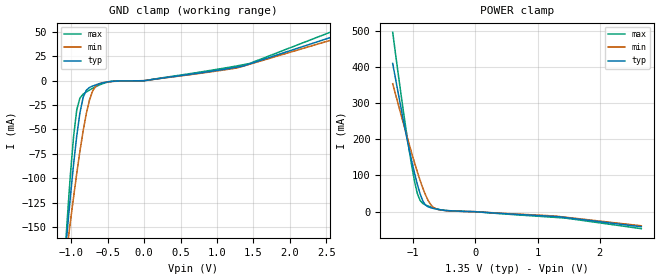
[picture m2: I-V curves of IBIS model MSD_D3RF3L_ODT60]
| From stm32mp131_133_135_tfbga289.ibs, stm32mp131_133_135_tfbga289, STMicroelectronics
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[Model] MSD_D3RF3L_ODT60
Model_type   Input
C_comp 2.201pF   2.154pF   2.263pF
Vinh = 810.000mV
Vinl = 540.000mV
[Receiver Thresholds]
Vth   =  0.675V
Vth_min  =  0.6615V
Vth_max  =  0.6885V
Vinh_ac  =  0.160V
Vinh_dc  =  0.090V
Vinl_ac  = -0.160V
Vinl_dc  = -0.090V
Tslew_ac =  5.000ns |Not specified, so set to high value
[Temperature Range]   25.000   125.000   -40.000
[Voltage Range]   1.350V   1.283V   1.450V
[GND Clamp Reference]   0.00V   0.00V   0.00V
[POWER Clamp Reference]   1.350V   1.283V   1.450V
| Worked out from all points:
|   GND clamp passes 1 mA (typ) near -0.48 V on its own axis
|   POWER clamp passes 1 mA (typ) near -0.20 V on its own axis
[GND Clamp]
-1.318V   -399.5mA   -339.2mA   -490.1mA
-1.098V   -193.9mA   -198.9mA   -195.7mA
-1.055V   -155.7mA   -171.8mA   -144.1mA
-1.011V   -119.5mA   -145.3mA   -97.39mA
-966.7mV  -86.12mA   -119.6mA   -57.63mA
-922.7mV  -56.68mA   -95.1mA    -29.86mA
-834.9mV  -17.04mA   -51.36mA   -13.76mA
-747mV    -6.894mA   -19.43mA   -9.56mA
-659.1mV  -4.192mA   -5.286mA   -6.03mA
-571.2mV  -2.301mA   -2.087mA   -3.13mA
1.45V     17.25mA    16.93mA    17.77mA
2.68V     47.37mA    44.21mA    53.39mA
[Power Clamp]
-1.33V    409.1mA    353.1mA    494.9mA
-1.155V   248.5mA    241.6mA    273.1mA
-1.023V   139mA      160.9mA    125.5mA
-978.8mV  106.2mA    135.2mA    83.6mA
-934.9mV  76.12mA    110.4mA    50.6mA
-890.9mV  49.81mA    87.04mA    31.29mA
-847mV    29.87mA    65.52mA    22.87mA
-803mV    18.41mA    46.44mA    18.65mA
-715.1mV  10.69mA    18.69mA    12.6mA
-583.3mV  5.781mA    5.363mA    5.989mA
1.438V    -15.9mA    -15.05mA   -17.61mA
2.668V    -41.64mA   -39mA      -46.87mA
